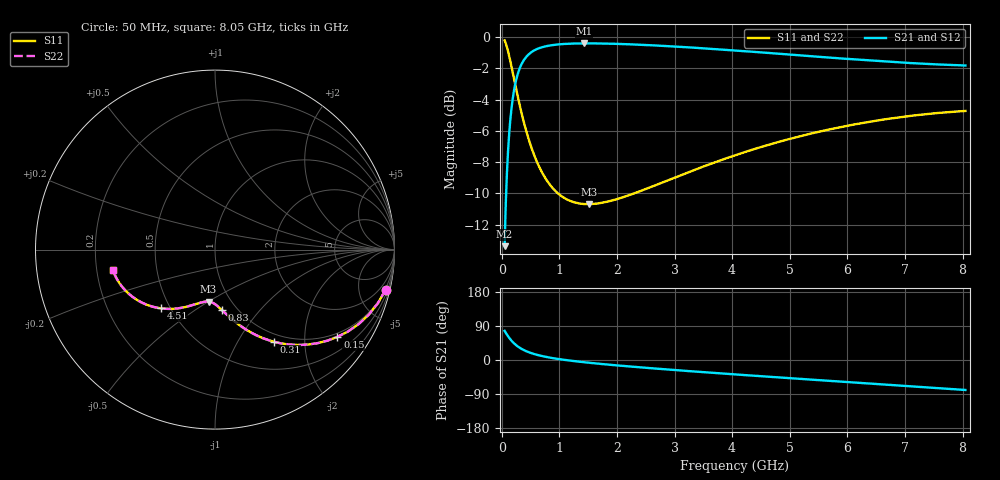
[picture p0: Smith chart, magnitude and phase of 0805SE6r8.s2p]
! AVX Thin Film Operation		Date: August 2001
! Description: Accu-P® Series, Thin Film, SMD, RF Capacitor
! Part Number: 08051J6R8BBT
! 50 MHz  -  8.05 GHz
! Serial Measurements
# mhz S db R 50
!	S11		S21		S12		S22
!	dB	Phase	dB	Phase	dB	Phase	dB	Phase
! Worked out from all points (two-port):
!   401 points, 50 MHz to 8.05 GHz, reference 50 ohm
!   highest |S21| = -0.39 dB at 1.43 GHz (marker M1); lowest = -13.4 dB at 50 MHz (marker M2)
!   |S21| within 3 dB of the highest: 214.1 MHz to end of sweep
!   lowest |S11| = -10.7 dB at 1.51 GHz (marker M3), VSWR 1.82, Z = 39.5 - j25 ohm
!   |S11| at or under -10 dB: 976 MHz to 2.3 GHz (1.324 GHz wide, 80.8 % of centre)
!   |S22| runs from -10.7 to -0.2 dB; largest |S21 - S12| = 0
!   S11 on the Smith chart (normalised r, x): 50 MHz: 0.88, -8.57; 150 MHz: 0.88, -2.88; 310 MHz: 0.88, -1.43; 830 MHz: 0.85, -0.65; 4.51 GHz: 0.44, -0.36; 8.05 GHz: 0.27, -0.09
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50  -0.20 -13.2  -13.38 76.8  -13.38 76.8  -0.20 -13.2
90  -0.63 -22.9  -8.73 67.1  -8.73 67.1  -0.63 -22.9
110  -0.90 -27.4  -7.27 62.6  -7.27 62.6  -0.90 -27.4
150  -1.54 -35.5  -5.26 54.5  -5.26 54.5  -1.54 -35.5
210  -2.60 -45.5  -3.47 44.5  -3.47 44.5  -2.60 -45.5
250  -3.31 -50.9  -2.74 39.1  -2.74 39.1  -3.31 -50.9
310  -4.32 -57.5  -2.01 32.5  -2.01 32.5  -4.32 -57.5
410  -5.80 -65.7  -1.33 24.3  -1.33 24.3  -5.80 -65.7
510  -7.01 -71.6  -0.97 18.3  -0.97 18.3  -7.01 -71.7
650  -8.29 -77.8  -0.70 12.2  -0.70 12.2  -8.29 -77.8
830  -9.42 -83.5  -0.53 6.4  -0.53 6.4  -9.42 -83.5
1090  -10.31 -89.6  -0.43 0.3  -0.43 0.3  -10.31 -89.7
1390  -10.67 -95.1  -0.39 -5.2  -0.39 -5.2  -10.67 -95.2
1430  -10.69 -95.8  -0.39 -5.9  -0.39 -5.9  -10.68 -95.8
1510  -10.69 -97.1  -0.39 -7.2  -0.39 -7.2  -10.69 -97.1
2070  -10.29 -105.0  -0.43 -15.1  -0.43 -15.1  -10.29 -105.1
2730  -9.39 -113.2  -0.54 -23.3  -0.54 -23.3  -9.39 -113.2
4050  -7.56 -127.9  -0.84 -38.0  -0.84 -38.0  -7.56 -127.9
4510  -7.02 -132.7  -0.97 -42.9  -0.97 -42.9  -7.02 -132.8
5390  -6.15 -141.8  -1.22 -51.9  -1.22 -51.9  -6.15 -141.8
6730  -5.22 -155.4  -1.57 -65.5  -1.57 -65.5  -5.21 -155.4
8050  -4.72 -169.0  -1.81 -79.1  -1.81 -79.1  -4.72 -169.0
